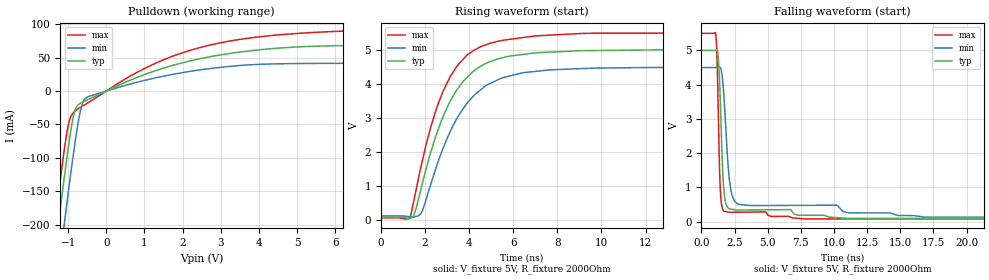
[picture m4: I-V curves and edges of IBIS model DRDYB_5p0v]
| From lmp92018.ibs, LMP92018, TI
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|   Model
[Model]   DRDYB_5p0v
Model_type   Open_drain
Polarity   Non-Inverting
Vmeas = 2.5
Vref = 5
Cref = 1pF
Rref = 2000
|   typ   min   max
C_comp   0.6389pF   0.6288pF   0.7669pF
[Voltage Range]   5   4.5   5.5
[Temperature Range]   27   125   -40
[Pullup Reference]   5   4.5   5.5
[Pulldown Reference]   0   0   0
[Power Clamp Reference]   5   4.5   5.5
[GND Clamp Reference]   0   0   0
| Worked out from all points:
|   slope of the pulldown table from 0 to 0.75 V, typ, clamps not added: 39.2 ohm
|   falling waveform, V_fixture 5V, R_fixture 2000Ohm: 20-80 % time 286ps typ, 487ps min, 198ps max; typ from 5 V to 0.089 V
|   rising waveform, V_fixture 5V, R_fixture 2000Ohm: 20-80 % time 1.8ns typ, 1.94ns min, 1.67ns max; typ from 0.089 V to 5 V
[Pulldown]
|   Voltage   I(typ)   I(min)   I(max)
-5V       -2.033A    -2.097A    -1.994A
-1.385V   -261.2mA   -332.4mA   -216.5mA
-1.235V   -190.9mA   -261.8mA   -146.9mA
-1.085V   -123.1mA   -192.6mA   -82.08mA
-965mV    -72.88mA   -138.9mA   -44.05mA
-845mV    -34.01mA   -88mA      -31.48mA
-755mV    -21.7mA    -53.71mA   -27.2mA
-635mV    -16.99mA   -20.54mA   -22.95mA
-515mV    -13.84mA   -9.673mA   -18.84mA
1.915V    41.12mA    26.77mA    55.72mA
4.645V    64.79mA    40.91mA    84.72mA
9.985V    69.31mA    45.95mA    93.78mA
[Ramp]
R_load = 2000
|   typ   min   max
dV/dt_r   2.94651/1.79404e-09   2.62531/1.93826e-09   3.25698/1.66338e-09
dV/dt_f   2.94651/2.86132e-10   2.62531/4.87025e-10   3.25698/1.97657e-10
[Falling Waveform]
V_fixture = 5V
V_fixture_min = 4.5V
V_fixture_max = 5.5V
R_fixture = 2000Ohm
C_fixture = 0F
|   Time   V(typ)   V(min)   V(max)
0s        5V         4.5V       5.5V
1.094ns   5.008V     4.5V       5.448V
1.245ns   4.907V     4.502V     3.723V
1.413ns   3.648V     4.507V     1.034V
1.644ns   1.191V     3.933V     328.2mV
2.081ns   371.8mV    1.328V     271.4mV
2.524ns   342.9mV    584.5mV    270.7mV
7.831ns   183.1mV    472.7mV    75.1mV
16.85ns   93.54mV    128.5mV    74.99mV
300ns     89.16mV    124.5mV    71.7mV
[Rising Waveform]
V_fixture = 5V
V_fixture_min = 4.5V
V_fixture_max = 5.5V
R_fixture = 2000Ohm
C_fixture = 0F
|   Time   V(typ)   V(min)   V(max)
0s        89.16mV    124.5mV    71.7mV
1.312ns   59.69mV    104.2mV    79.45mV
1.48ns    120.5mV    95.9mV     533.6mV
1.821ns   930.1mV    202mV      1.58V
2.516ns   2.515V     1.559V     3.263V
3.115ns   3.452V     2.556V     4.173V
3.827ns   4.133V     3.358V     4.789V
5.476ns   4.753V     4.166V     5.266V
9.108ns   4.966V     4.441V     5.47V
300ns     5V         4.5V       5.5V
